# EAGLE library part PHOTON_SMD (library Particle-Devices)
Particle Photon (without headers) WiFi development board footprint - designed to be surface mounted with 7 extra exposed pads on the bottom of the board which include, 3 RGB LED outputs, /SETUP, EN (3.3V SMPS enable input), USB D+ and USB D-. Product datasheet: here Design files: here Github : Particle devices library
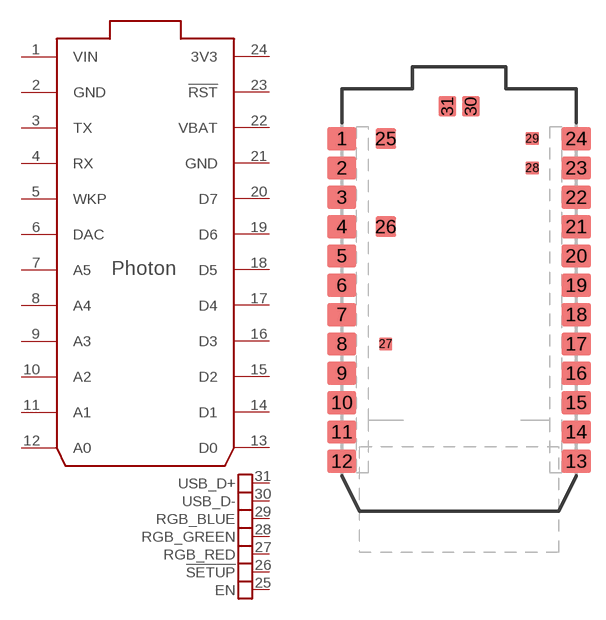
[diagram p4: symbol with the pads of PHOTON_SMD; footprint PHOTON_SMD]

Designator prefix -; gates G$1=PHOTON G$2=PHOTON_PADS

## PHOTON_SMD  [PHOTON_SMD]
1  G$1:VIN  pwr
2  G$1:GND  pwr
3  G$1:TX
4  G$1:RX
5  G$1:WKP
6  G$1:DAC
7  G$1:A5
8  G$1:A4
9  G$1:A3
10  G$1:A2
11  G$1:A1
12  G$1:A0
13  G$1:D0
14  G$1:D1
15  G$1:D2
16  G$1:D3
17  G$1:D4
18  G$1:D5
19  G$1:D6
20  G$1:D7
21  G$1:GND  pwr
22  G$1:VBAT  pwr
23  G$1:!RST
24  G$1:3V3  pwr
25  G$2:EN
26  G$2:!SETUP
27  G$2:RGB_RED
28  G$2:RGB_GREEN
29  G$2:RGB_BLUE
30  G$2:USB_D-
31  G$2:USB_D+

## Footprint PHOTON_SMD (pad centres in mm)
smd 2.54 x 2.032: 1 0,33.02; 2 0,30.48; 3 0,27.94; 4 0,25.4; 5 0,22.86; 6 0,20.32; 7 0,17.78; 8 0,15.24; 9 0,12.7; 10 0,10.16; 11 0,7.62; 12 0,5.08; 13 20.32,5.08; 14 20.32,7.62; 15 20.32,10.16; 16 20.32,12.7; 17 20.32,15.24; 18 20.32,17.78; 19 20.32,20.32; 20 20.32,22.86; 21 20.32,25.4; 22 20.32,27.94; 23 20.32,30.48; 24 20.32,33.02
smd 1.778 x 1.778: 25 3.81,33.02; 26 3.81,25.4
smd 1.143 x 1.143: 27 3.81,15.24; 28 16.51,30.48; 29 16.51,33.02
smd 1.524 x 1.778: 30 11.176,35.814; 31 9.144,35.814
